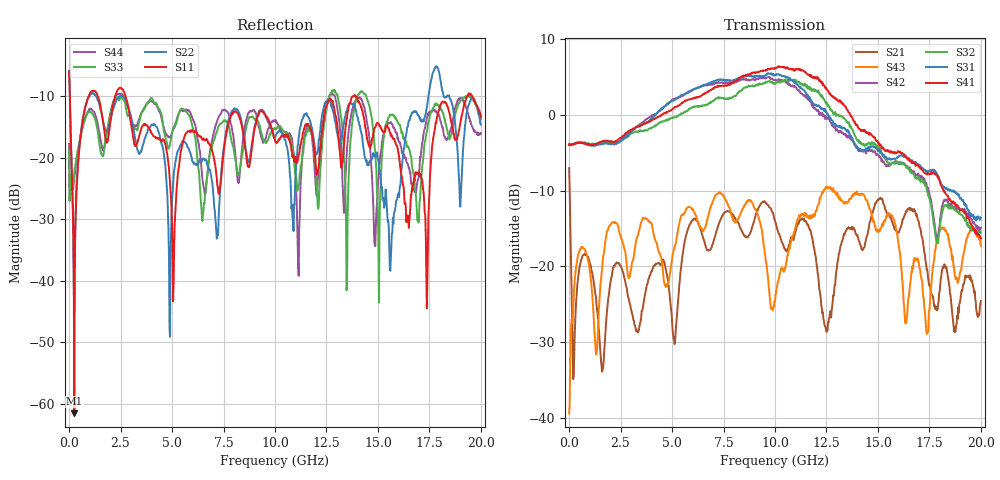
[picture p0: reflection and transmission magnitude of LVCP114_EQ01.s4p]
!Agilent Technologies,N5230A,MY46400459,A.07.50.48
!Agilent N5230A: A.07.50.48
!Date: Monday, January 09, 2012 14:00:46
!Correction: S11(Full 4 Port(1,2,3,4))
!S12(Full 4 Port(1,2,3,4))
!S13(Full 4 Port(1,2,3,4))
!S14(Full 4 Port(1,2,3,4))
!S21(Full 4 Port(1,2,3,4))
!S22(Full 4 Port(1,2,3,4))
!S23(Full 4 Port(1,2,3,4))
!S24(Full 4 Port(1,2,3,4))
!S31(Full 4 Port(1,2,3,4))
!S32(Full 4 Port(1,2,3,4))
!S33(Full 4 Port(1,2,3,4))
!S34(Full 4 Port(1,2,3,4))
!S41(Full 4 Port(1,2,3,4))
!S42(Full 4 Port(1,2,3,4))
!S43(Full 4 Port(1,2,3,4))
!S44(Full 4 Port(1,2,3,4))
!S4P File: Measurements: <S11,S12,S13,S14>,
!<S21,S22,S23,S24>,
!<S31,S32,S33,S34>,
!<S41,S42,S43,S44>:
# Hz S  dB  R 50
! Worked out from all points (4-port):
!   801 points, 300 kHz to 20 GHz, reference 50 ohm
!   strongest paths, dB at 300 kHz, 5 GHz, 10 GHz, 15 GHz, 20 GHz:
!     S41: -4.0, 0.7, 6.1, -3.6, -16.3
!     S31: -4.0, 1.9, 5.2, -4.8, -13.6
!     S32: -3.8, -0.4, 4.1, -4.4, -15.5
!     S42: -3.9, 1.9, 4.6, -5.3, -14.9
!     S43: -39.4, -19.0, -24.6, -15.2, -17.3
!     S21: -7.0, -27.2, -14.0, -11.3, -24.6
!   lowest |S11| = -61.6 dB at 250.3 MHz (marker M1), VSWR 1.00, Z = 50.1 - j0.0024 ohm
!   |S11| at or under -10 dB: 34.43 MHz to 955.3 MHz (920.8 MHz wide, 186 % of centre); 2.738 GHz to 13.81 GHz (11.07 GHz wide, 134 % of centre); 13.91 GHz to 19.36 GHz (5.456 GHz wide, 32.8 % of centre)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
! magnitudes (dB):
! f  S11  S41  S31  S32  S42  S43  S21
! 300 kHz  -6.0  -4.0  -4.0  -3.8  -3.9  -39.4  -7.0
! 250.3 MHz  -61.6  -3.9  -3.9  -3.8  -3.8  -22.6  -31.4
! 1.15 GHz  -9.2  -4.0  -4.1  -3.8  -4.0  -24.7  -21.3
! 4.9 GHz  -24.1  0.5  1.7  -0.5  1.7  -20.9  -24.3
! 13.88 GHz  -9.8  -0.9  -3.8  -2.7  -4.0  -10.3  -15.2
! 17.38 GHz  -44.5  -7.9  -7.6  -10.0  -9.4  -28.9  -20.5
! 20 GHz  -13.4  -16.3  -13.6  -15.5  -14.9  -17.3  -24.6
